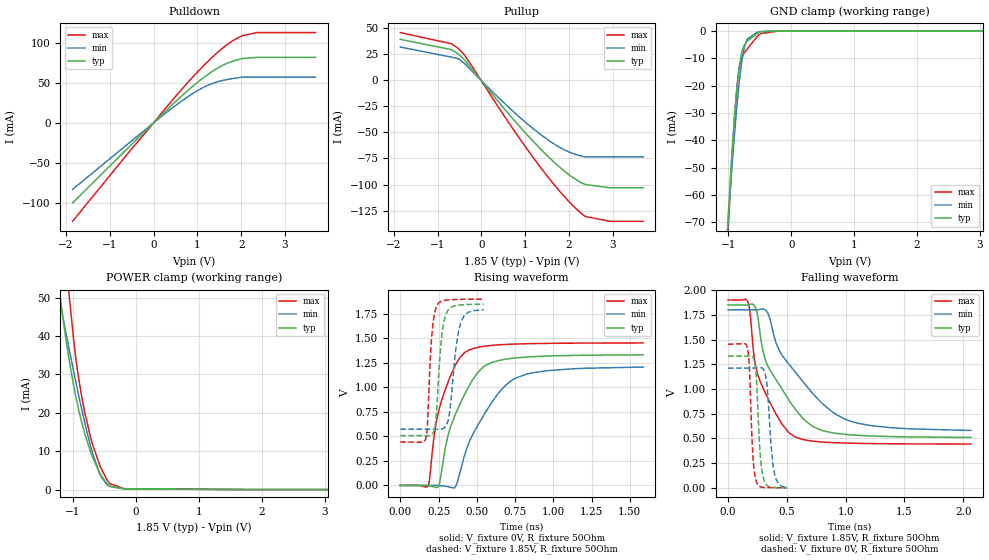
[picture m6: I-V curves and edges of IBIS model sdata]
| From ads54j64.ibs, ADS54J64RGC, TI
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|   sdata Model
[Model]   sdata
Model_type   I/O
Polarity   Non-Inverting
Enable   Active-High
Vinl = 0.555
Vinh = 1.295
Vmeas = 0.925
Vref = 0
Cref = 2pF
Rref = 50
|   typ   min   max
|   (nom PVT)   (fast PVT)   (slow PVT)
C_comp   4.830e-13   4.319e-13   5.507e-13
| Where nom  PVT is Nominal Process, 1.85V, 27C
|   Fast PVT is Strong Process,  1.9V, -40C
|   Slow PVT is Weak Process,   1.8V, 125C
[Voltage Range]   1.85   1.8   1.9
|Junction Temperature
[Temperature Range]   27   125   -40
[Pullup Reference]   1.85   1.8   1.9
[Pulldown Reference]   0   0   0
[Power Clamp Reference]   1.85   1.8   1.9
[GND Clamp Reference]   0   0   0
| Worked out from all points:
|   slope of the pulldown table from 0 to 0.278 V, typ, clamps not added: 18.7 ohm
|   slope of the pullup table from 0 to 0.278 V, typ, clamps not added: 19.2 ohm
|   GND clamp passes 1 mA (typ) near -0.54 V on its own axis
|   POWER clamp passes 1 mA (typ) near -0.42 V on its own axis
|   falling waveform, V_fixture 1.85V, R_fixture 50Ohm: 20-80 % time 312ps typ, 442ps min, 214ps max; typ from 1.85 V to 0.511 V
|   rising waveform, V_fixture 0V, R_fixture 50Ohm: 20-80 % time 186ps typ, 246ps min, 135ps max; typ from 0 V to 1.33 V
|   rising waveform, V_fixture 1.85V, R_fixture 50Ohm: 20-80 % time 38ps typ, 50.4ps min, 29.7ps max; typ from 0.508 V to 1.85 V
|   falling waveform, V_fixture 0V, R_fixture 50Ohm: 20-80 % time 36.1ps typ, 44.6ps min, 29.9ps max; typ from 1.33 V to 0.002 V
[Pulldown]
|   Voltage   I(typ)   I(min)   I(max)
-1.85V    -99.59mA   -82.68mA   -122.4mA
-490.3mV  -26.03mA   -21.75mA   -31.48mA
584.6mV   30.76mA    25.05mA    38.19mA
901.2mV   45.95mA    36.81mA    57.49mA
1.184V    58.19mA    45.48mA    73.61mA
1.431V    67.3mA     50.81mA    86.4mA
1.648V    73.48mA    53.71mA    96.2mA
1.844V    77.45mA    55.57mA    103.4mA
2.037V    80.28mA    57.08mA    108.8mA
2.362V    81.63mA    57.08mA    112.5mA
3.7V      81.63mA    57.08mA    112.5mA
[GND Clamp]
|   Voltage   I(typ)   I(min)   I(max)
-1.85V    -493.1mA   -441.4mA   -539.3mA
-1.015V   -72.61mA   -73.55mA   -77.35mA
-957mV    -49.51mA   -54.05mA   -52.03mA
-901.9mV  -30.91mA   -37.45mA   -31.65mA
-860.2mV  -19.94mA   -26.35mA   -19.69mA
-821.4mV  -12.4mA    -17.48mA   -12.54mA
-775.4mV  -6.819mA   -9.431mA   -9.166mA
-746.6mV  -5.152mA   -6.02mA    -8.081mA
-705.2mV  -3.892mA   -3.174mA   -6.72mA
-541.4mV  -939.8uA   -471.1uA   -2.057mA
-185mV    -17.51uA   -15.43uA   -21.46uA
3.7V      0A         0A         0A
[Pullup]
|   Voltage   I(typ)   I(min)   I(max)
-1.85V    39.27mA    31.91mA    45.76mA
-675.8mV  29.33mA    22.12mA    34.96mA
-483.8mV  23.75mA    19.53mA    28.79mA
-381.3mV  19.52mA    15.97mA    24.07mA
494.6mV   -25.72mA   -20.7mA    -32.31mA
1.147V    -56.83mA   -45.09mA   -71.82mA
1.728V    -80.96mA   -62.74mA   -103.3mA
2.034V    -91.5mA    -69.35mA   -117.7mA
2.267V    -97.94mA   -72.63mA   -127.2mA
2.393V    -100mA     -73.52mA   -130.8mA
2.94V     -103.1mA   -73.52mA   -135.2mA
3.7V      -103.1mA   -73.52mA   -135.2mA
[POWER Clamp]
|   Voltage   I(typ)   I(min)   I(max)
-1.85V    203.1mA    123.3mA    310.8mA
-1.28V    61.27mA    55.34mA    104.3mA
-1.206V   50.4mA     48.77mA    83.2mA
-1.058V   33.43mA    36.29mA    50.04mA
-987.4mV  26.87mA    30.55mA    38.5mA
-949mV    23.71mA    27.52mA    33.39mA
-810.7mV  14.42mA    17.23mA    19.84mA
-698mV    8.804mA    9.947mA    12.24mA
-577mV    4.343mA    4.149mA    6.411mA
-413.6mV  946.7uA    795uA      1.568mA
-185mV    197.8uA    182uA      240.2uA
3.7V      0A         0A         0A
[Ramp]
R_load = 50
|   typ   min   max
dV/dt_r   0.799474/1.8695e-10   0.727094/2.48707e-10   0.871468/1.35264e-10
dV/dt_f   0.805352/3.13752e-10   0.736463/4.47153e-10   0.874231/2.14549e-10
[Falling Waveform]
V_fixture = 1.85V
V_fixture_min = 1.8V
V_fixture_max = 1.9V
R_fixture = 50Ohm
|   Time   V(typ)   V(min)   V(max)
0s        1.85V      1.8V       1.9V
170.6ps   1.85V      1.8V       1.876V
192.5ps   1.856V     1.8V       1.718V
229.3ps   1.834V     1.799V     1.269V
325.7ps   1.268V     1.79V      940.3mV
433.8ps   1.048V     1.394V     694.9mV
570.9ps   797mV      1.173V     516.3mV
731.6ps   614.5mV    940.2mV    471.7mV
1.057ns   535.5mV    668.6mV    451.9mV
2.065ns   510.5mV    581.8mV    443.7mV
[Rising Waveform]
V_fixture = 0V
V_fixture_min = 0V
V_fixture_max = 0V
R_fixture = 50Ohm
|   Time   V(typ)   V(min)   V(max)
0s        86.46nV    542.2nV    588.8nV
182ps     -2.706mV   -46.27uV   -4.452mV
224.2ps   -16.79mV   453.1uV    539.8mV
258.2ps   36.18mV    -1.652mV   801.2mV
312ps     508.5mV    -13.31mV   1.051V
356.6ps   710.2mV    -21.76mV   1.214V
428.1ps   951.8mV    346.9mV    1.362V
548.5ps   1.213V     723.1mV    1.418V
756.7ps   1.3V       1.096V     1.441V
1.588ns   1.331V     1.206V     1.452V
[Rising Waveform]
V_fixture = 1.85V
V_fixture_min = 1.8V
V_fixture_max = 1.9V
R_fixture = 50Ohm
|   Time   V(typ)   V(min)   V(max)
0s        507.7mV    572.5mV    442.9mV
166.8ps   507.2mV    572.5mV    475.9mV
177.2ps   506.2mV    572.5mV    609mV
206.6ps   519.3mV    572.8mV    1.541V
227.1ps   597.8mV    572.5mV    1.772V
240.5ps   841.2mV    571.7mV    1.834V
272.3ps   1.537V     574.8mV    1.879V
306.9ps   1.773V     635.7mV    1.889V
395.4ps   1.839V     1.657V     1.896V
545.4ps   1.847V     1.79V      1.899V
[Falling Waveform]
V_fixture = 0V
V_fixture_min = 0V
V_fixture_max = 0V
R_fixture = 50Ohm
|   Time   V(typ)   V(min)   V(max)
0s        1.332V     1.212V     1.452V
166.1ps   1.332V     1.212V     1.407V
182ps     1.335V     1.212V     1.216V
222.1ps   1.291V     1.211V     186.5mV
241.3ps   1.108V     1.212V     63.75mV
273.5ps   348.7mV    1.216V     12.01mV
304.9ps   84.54mV    1.189V     5.237mV
332.2ps   25.29mV    1.032V     4.338mV
393ps     5.005mV    158.9mV    2.465mV
499.2ps   2.329mV    6.098mV    1.031mV
